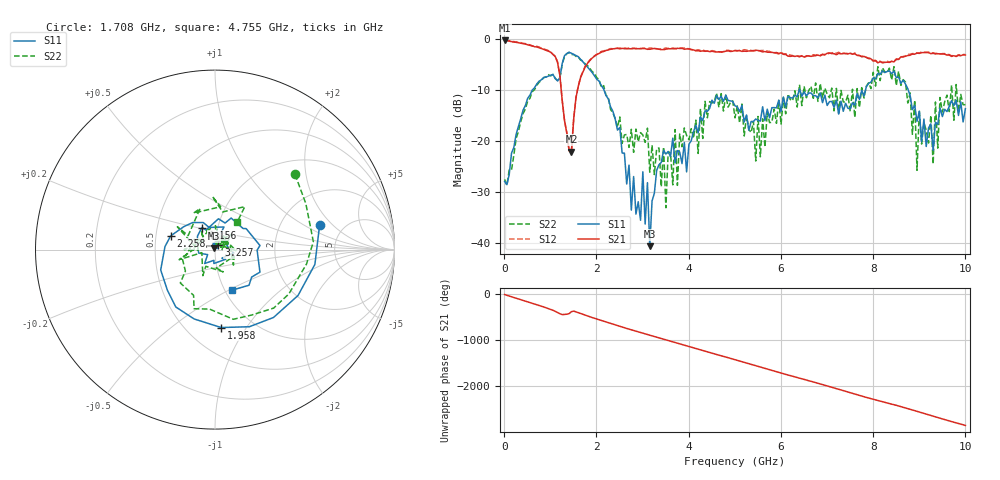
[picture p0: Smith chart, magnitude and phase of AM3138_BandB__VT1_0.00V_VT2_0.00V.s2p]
! Date/Time: Tue, Nov 13, 2018 4:39 PM
! Network Analyzer: Agilent Technologies E8364B Rev: A.07.50.67
! Sweep from 0.010 to 10.000 GHz, 201 Points, Sweep Type: LIN
! Power Supply: -0.000 V, 0.000 A
# Hz S DB R 50
!freq MagS11 AngS11 MagS21 AngS21 MagS12 AngS12 MagS22 AngS22
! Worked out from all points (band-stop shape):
!   201 points, 10 MHz to 10 GHz, reference 50 ohm
!   highest |S21| = -0.27 dB at 10 MHz (marker M1); lowest = -22.1 dB at 1.459 GHz (marker M2)
!   |S21| within 3 dB of the highest: start of sweep to 1.088 GHz; 1.971 GHz to 6.144 GHz (4.172 GHz wide, 103 % of centre)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
!   lowest |S11| = -40.7 dB at 3.157 GHz (marker M3), VSWR 1.02, Z = 49.5 + j0.788 ohm
!   |S11| at or under -10 dB: 2.165 GHz to 6.396 GHz (4.231 GHz wide, 98.8 % of centre); 6.411 GHz to 7.834 GHz (1.423 GHz wide, 20 % of centre); 8.761 GHz to end of sweep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
!   |S22| runs from -33.1 to -2.6 dB; largest |S21 - S12| = 0.033
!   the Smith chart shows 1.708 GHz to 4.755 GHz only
!   S11 on the Smith chart (normalised r, x): 1.708 GHz: 3.34, +1.40; 1.958 GHz: 0.72, -0.77; 2.258 GHz: 0.60, +0.10; 3.257 GHz: 1.04, +0.05; 4.156 GHz: 0.84, +0.21; 4.755 GHz: 1.08, -0.52
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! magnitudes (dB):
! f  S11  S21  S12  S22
! 10 MHz  -27.9  -0.3  -0.3  -27.5
! 1.109 GHz  -7.8  -3.4  -3.4  -7.7
! 1.459 GHz  -2.8  -22.1  -22.0  -3.1
! 1.708 GHz  -4.5  -6.4  -6.3  -4.3
! 1.958 GHz  -7.2  -3.4  -3.3  -6.7
! 2.258 GHz  -11.7  -2.1  -2.1  -11.4
! 2.757 GHz  -33.6  -1.9  -1.8  -17.7
! 3.107 GHz  -28.2  -2.0  -1.9  -17.5
! 3.157 GHz  -40.7  -2.0  -1.8  -26.1
! 3.257 GHz  -30.3  -1.8  -1.9  -26.6
! 3.357 GHz  -24.7  -2.0  -2.0  -21.4
! 3.507 GHz  -22.6  -2.0  -1.8  -33.1
! 4.156 GHz  -16.9  -2.3  -2.2  -15.9
! 4.755 GHz  -12.2  -2.5  -2.4  -14.1
! 5.005 GHz  -13.1  -2.2  -2.3  -15.5
! 6.703 GHz  -11.1  -3.3  -3.1  -11.6
! 8.352 GHz  -6.2  -4.6  -4.5  -5.7
! 8.901 GHz  -13.0  -3.0  -2.9  -12.0
! 8.951 GHz  -16.2  -2.8  -2.7  -25.8
! 9.001 GHz  -14.2  -2.8  -2.7  -14.0
! 9.301 GHz  -21.9  -2.8  -2.7  -24.5
! 10 GHz  -13.7  -3.1  -3.0  -12.9
